FUNCTION_BLOCK "Main"
VERSION : 0.1
   VAR_INPUT
      in1 : Bool;
      in2 : Bool;
      in3 : Bool;
   END_VAR

   VAR_OUTPUT
      out1 : Bool;
   END_VAR


BEGIN
NETWORK
TITLE =
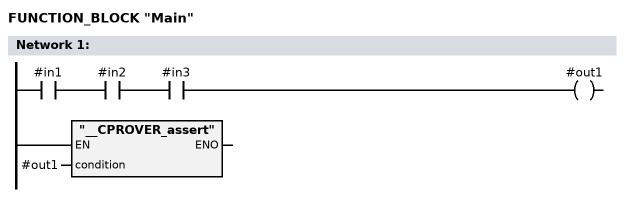
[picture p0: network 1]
      A #in1;
      A #in2;
      A #in3;
      = #out1;
      CALL "__CPROVER_assert"
      (  condition := #out1
      );

END_FUNCTION_BLOCK

